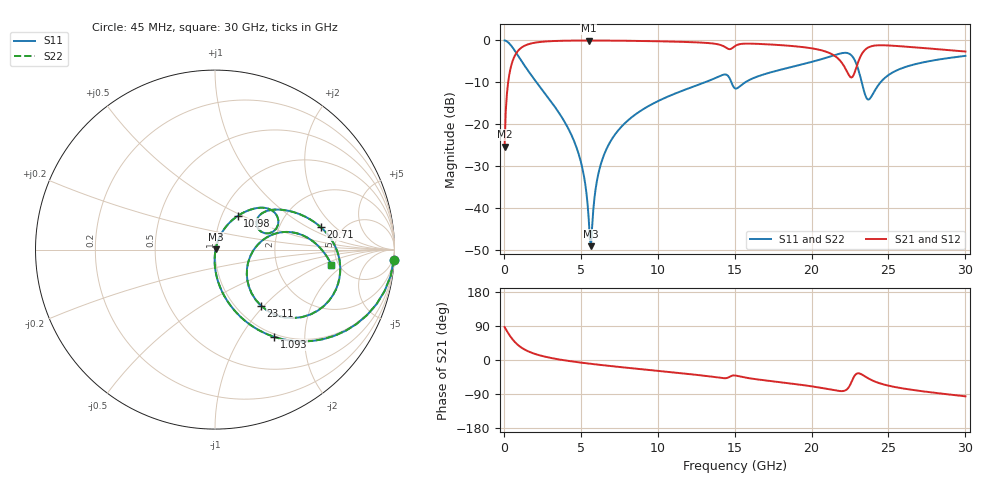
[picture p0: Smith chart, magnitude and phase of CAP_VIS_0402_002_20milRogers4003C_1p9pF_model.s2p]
! S-parameter model data by Modelithics Inc.  support@modelithics.com  813-866-6335  Tampa FL USA
! S-Parameter data specifications:
! Substrate: 20-mil Rogers 4003C, substrate thickness, H=0.508mm, Dielectric constant, Er=3.75
! PCB Mounting Pad Footprint: Pad width, PadW=0.50mm , Pad length, PadL=0.50mm , Pad gap, PadG (edge-to-edge)=0.40mm , Reference planes=1.4mm apart
! Created Wed Nov 18 12:43:25 2015
# hz S ma R 50
! 2 Port Network Data from SP1.SP block
! freq  magS11  angS11  magS21  angS21  magS12  angS12  magS22  angS22
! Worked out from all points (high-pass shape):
!   401 points, 45 MHz to 30 GHz, reference 50 ohm
!   highest |S21| = -0.03 dB at 5.512 GHz (marker M1); lowest = -25.3 dB at 45 MHz (marker M2)
!   |S21| within 3 dB of the highest: 806.2 MHz to 21.18 GHz (20.37 GHz wide, 185 % of centre); 23.3 GHz to end of sweep
!   lowest |S11| = -49.0 dB at 5.662 GHz (marker M3), VSWR 1.01, Z = 50.4 + j0.0598 ohm
!   |S11| at or under -10 dB: 2.125 GHz to 13.05 GHz (10.92 GHz wide, 144 % of centre); 14.79 GHz to 15.68 GHz (888.3 MHz wide, 5.83 % of centre); 23.26 GHz to 24.48 GHz (1.215 GHz wide, 5.09 % of centre)
!   |S22| runs from -49.0 to 0.0 dB; largest |S21 - S12| = 0
!   S11 on the Smith chart (normalised r, x): 45 MHz: 1, -36; 1.093 GHz: 0.96, -1.42; 10.98 GHz: 1.19, +0.47; 20.71 GHz: 3.47, +1.35; 23.11 GHz: 1.28, -0.96; 30 GHz: 4.39, -1.29
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4.5e7  0.9985 -3.2  0.05451 86.8  0.05451 86.8  0.9985 -3.2
4.194375e8  0.8901 -27.8  0.4553 62.1  0.4553 62.1  0.8901 -27.8
1.093425e9  0.5871 -55.9  0.8083 34.0  0.8083 34.0  0.5871 -55.9
2.066962e9  0.3268 -74.3  0.9432 15.4  0.9432 15.4  0.3268 -74.3
3.93915e9  0.1076 -89.4  0.9913 -0.8  0.9913 -0.8  0.1076 -89.4
5.062462e9  0.03228 -91.6  0.9962 -7.2  0.9962 -7.2  0.03228 -91.6
5.511788e9  0.007563 -73.6  0.9965 -9.4  0.9965 -9.4  0.007563 -73.6
5.661562e9  0.003554 9.6  0.9965 -10.1  0.9965 -10.1  0.003554 9.6
6.185775e9  0.02807 70.2  0.9959 -12.6  0.9959 -12.6  0.02807 70.2
6.859762e9  0.05972 70.8  0.9943 -15.6  0.9943 -15.6  0.05972 70.8
1.007992e10  0.1919 59.5  0.976 -29.0  0.976 -29.0  0.1919 59.5
1.097858e10  0.227 55.9  0.9678 -32.6  0.9678 -32.6  0.227 55.9
1.427362e10  0.3908 31.9  0.8545 -48.1  0.8545 -48.1  0.3908 31.9
1.50225e10  0.2684 24.6  0.8578 -40.9  0.8578 -40.9  0.2684 24.6
2.003996e10  0.5571 17.5  0.8032 -69.7  0.8032 -69.7  0.5571 17.5
2.071395e10  0.603 11.9  0.756 -74.1  0.756 -74.1  0.603 11.9
2.22117e10  0.7116 -15.5  0.4584 -79.9  0.4584 -79.9  0.7116 -15.5
2.266102e10  0.6422 -34.3  0.3681 -52.0  0.3681 -52.0  0.6422 -34.3
2.311035e10  0.4053 -50.7  0.6024 -35.5  0.6024 -35.5  0.4053 -50.7
2.370945e10  0.1977 -15.5  0.8283 -49.0  0.8283 -49.0  0.1977 -15.5
2.505742e10  0.3933 14.4  0.8695 -68.2  0.8695 -68.2  0.3933 14.4
3e10  0.6543 -7.4  0.7372 -95.8  0.7372 -95.8  0.6543 -7.4
